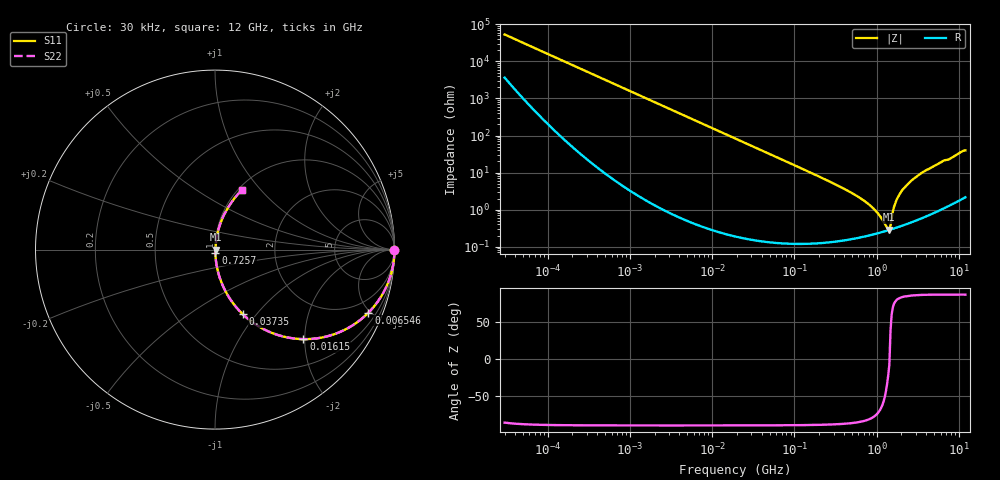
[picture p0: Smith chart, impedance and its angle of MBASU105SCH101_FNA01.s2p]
! MBASU105SCH101_FNA01  S-PARAMETER MODEL  ( General Type )
! Model Generated by TAIYO YUDEN Corporation (http://www.ty-top.com)
! Version 1.0
! TAIYO YUDEN Control No. 130207
! Copyright(c) 2013 TAIYO YUDEN CO.,LTD. All Rights Reserved.
! Product Description (link to TY-COMPAS)
! https://ds.yuden.co.jp/TYCOMPAS/or/detail?pn=MBASU105SCH101JFNA01&u=M
! Products Name : Multilayer Ceramic Capacitors
! Characteristics :
!  Capacitance : 100 pF , Rated Voltage : 50V , TCC : CH / C0H
!  Case Size : 1.0 x 0.5 / 0.039 x 0.02 [mm/inch] , Thickness : 0.5 / 0.02 [mm/inch]
!  (Conditions: Temperature = 25 degC , DC Bias Current/Voltage = 0A / 0V)
! External Node Assignments :
!  1  o---| |---o  2
! GND o---------o GND
! Frequency Range : 30000Hz  -  12GHz  [ 401 STEP ]
# MHz S RI R 50
! Freq[MHz].  S11 Real  S11 Imag  S21 Real  S21 Imag  S12 Real  S12 Imag  S22 Real  S22 Imag
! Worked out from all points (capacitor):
!   401 points, 30 kHz to 12 GHz, reference 50 ohm
!   read as one part in series: C = 100 pF near 32 kHz
!   lowest |Z| = 286 mohm at 1.428 GHz (marker M1)
!   series resonance near 1.435 GHz, so ESL is about 120 pH
!   S11 on the Smith chart (normalised r, x): 30 kHz: open; 6.546 MHz: 1.01, -4.86; 16.15 MHz: 1.00, -1.97; 37.35 MHz: 1.00, -0.85; 725.7 MHz: 1.00, -0.03; 12 GHz: 1.04, +0.79
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0.03  0.9999 -0.00188  0.000133 0.00188  0.000133 0.00188  0.9999 -0.00188
0.260295  0.9997 -0.0164  0.000347 0.0164  0.000347 0.0164  0.9997 -0.0164
2.258455  0.98 -0.1391  0.02 0.1391  0.02 0.1391  0.98 -0.1391
6.54608  0.8547 -0.3516  0.1453 0.3516  0.1453 0.3516  0.8547 -0.3516
16.14825  0.4923 -0.4989  0.5077 0.4989  0.5077 0.4989  0.4923 -0.4989
18.97367  0.4128 -0.4912  0.5872 0.4912  0.5872 0.4912  0.4128 -0.4912
37.34732  0.1542 -0.3594  0.8458 0.3594  0.8458 0.3594  0.1542 -0.3594
68.9219  0.0514 -0.2181  0.9486 0.2181  0.9486 0.2181  0.0514 -0.2181
164.6252  0.0102 -0.0943  0.9898 0.0943  0.9898 0.0943  0.0102 -0.0943
419.4166  0.0027 -0.0346  0.9973 0.0346  0.9973 0.0346  0.0027 -0.0346
725.66  0.00217 -0.0164  0.9978 0.0164  0.9978 0.0164  0.00217 -0.0164
1001.808  0.00233 -0.00834  0.9977 0.00834  0.9977 0.00834  0.00233 -0.00834
1339.156  0.00272 -0.00184  0.9973 0.00184  0.9973 0.00184  0.00272 -0.00184
1428.372  0.00283 -0.000365  0.9972 0.000365  0.9972 0.000365  0.00283 -0.000365
1475.185  0.0029 0.00227  0.9971 -0.00227  0.9971 -0.00227  0.0029 0.00227
1678.29  0.00337 0.014  0.9966 -0.014  0.9966 -0.014  0.00337 0.014
1790.1  0.00373 0.02  0.9963 -0.02  0.9963 -0.02  0.00373 0.02
2036.564  0.00473 0.0326  0.9953 -0.0326  0.9953 -0.0326  0.00473 0.0326
2471.32  0.00695 0.0516  0.993 -0.0516  0.993 -0.0516  0.00695 0.0516
3881.513  0.0184 0.1087  0.9816 -0.1087  0.9816 -0.1087  0.0184 0.1087
7640.278  0.0608 0.2128  0.9392 -0.2128  0.9392 -0.2128  0.0608 0.2128
12000  0.1488 0.3297  0.8512 -0.3297  0.8512 -0.3297  0.1488 0.3297
